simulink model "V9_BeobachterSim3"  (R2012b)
settings: Solver=ode4  SolverMode=SingleTasking  StartTime=0.0  StopTime=3  FixedStep=0.001  RelTol=1e-3
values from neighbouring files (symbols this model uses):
  A = [-2 1    [V9_1_Beobachterdesign.m]    (also in V9_2_Beobachterdesign.m; V9_3_Beobachterdesign.m)
  Ad = expm(A*Ts)    [V9_3_Beobachterdesign.m]
  B = [1; 1]    [V9_1_Beobachterdesign.m]    (also in V9_2_Beobachterdesign.m = [0; 1]; V9_3_Beobachterdesign.m = [0; 1])
  Bd = (Ad-eye(2))*inv(A)*B    [V9_3_Beobachterdesign.m]
  C = [1 0]    [V9_1_Beobachterdesign.m]    (also in V9_2_Beobachterdesign.m; V9_3_Beobachterdesign.m; LinProb.m = LinProb(A.GetSize()))
  Gd = acker(Ad',C',poles)    [V9_3_Beobachterdesign.m]
  K = place(A,B,pc)    [V9_2_Beobachterdesign.m]    (also in V9_3_Beobachterdesign.m = place(Ad,Bd,pcd); kalman1.m = sys(2)/(sigma*sigma); kalman2.m = sys(2)/(sigma*sigma); kalman3.m = sys(2)/(r2))
  Ts = 0.01    [V9_3_Beobachterdesign.m]    (also in V2_4_tdomain.m = 0.1; V2_6_UTFDiskretizierung.m = 0.1; V2_7_multiZ.m = 0.1)

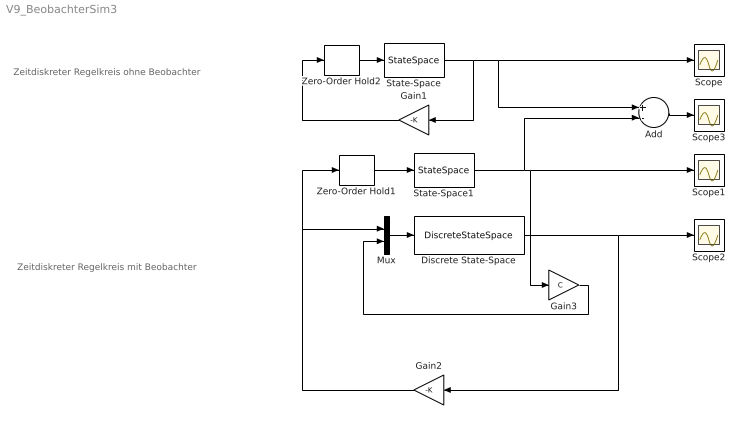
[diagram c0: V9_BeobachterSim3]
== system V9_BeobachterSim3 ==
  note: Zeitdiskreter Regelkreis ohne Beobachter
  note: Zeitdiskreter Regelkreis mit Beobachter
  Add : Sum  Inputs=+-
  Discrete State-Space : DiscreteStateSpace  A=Ad-Gd'*C  B=[Bd Gd']  C=eye(2)  D=zeros(2,2)  X0=[0;0]  SampleTime=Ts
  Gain1 : Gain  Gain=-K  Multiplication=Matrix(K*u)
  Gain2 : Gain  Gain=-K  Multiplication=Matrix(K*u)
  Gain3 : Gain  Gain=C  Multiplication=Matrix(K*u)
  Mux : Mux  Inputs=2
  Scope{,1..3} (4 alike) : Scope
  State-Space : StateSpace  A=A  B=B  C=eye(2)  D=[0; 0]  X0=[2; 1]
  State-Space1 : StateSpace  A=A  B=B  C=eye(2)  D=[0; 0]  X0=[2; 1]
  Zero-Order Hold1 : ZeroOrderHold  SampleTime=Ts
  Zero-Order Hold2 : ZeroOrderHold  SampleTime=Ts
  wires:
  Gain3/1 -> Mux/2
  State-Space/1 -> Gain1/1, Scope/1, Add/1
  State-Space1/1 -> Gain3/1, Scope1/1, Add/2
  Add/1 -> Scope3/1
  Discrete State-Space/1 -> Gain2/1, Scope2/1
  Gain1/1 -> Zero-Order Hold2/1
  Gain2/1 -> Mux/1, Zero-Order Hold1/1
  Zero-Order Hold1/1 -> State-Space1/1
  Mux/1 -> Discrete State-Space/1
  Zero-Order Hold2/1 -> State-Space/1
